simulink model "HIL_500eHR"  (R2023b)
settings: Solver=VariableStepAuto  StartTime=0.0  StopTime=Time  RelTol=1e-3
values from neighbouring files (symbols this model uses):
  BEV_mot = load("20241002_EM_Polito_Maps.mat")    [Init_FWD_500eHR.m]
undefined symbols (not defined in the file or in its folder): battery350V, bevGear, flip, motorDrive, T_EM_max, T_EM_max_cont, vehicle
libraries: fl_lib x38, nesl_utility x25, sdl_lib x11, slpidlib x3, simulink x3, ee_lib x2
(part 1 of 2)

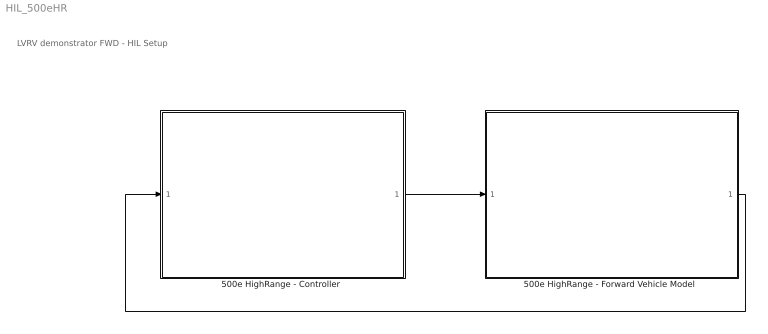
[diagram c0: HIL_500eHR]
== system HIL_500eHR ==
  note: LVRV demonstrator FWD - HIL Setup
  "500e HighRange - Controller " : Subsystem
  "500e HighRange - Forward Vehicle Model " : Subsystem
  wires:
  "500e HighRange - Forward Vehicle Model "/1(Bus Element Out) -> "500e HighRange - Controller "/1(BusElementIn)
  "500e HighRange - Controller "/1(Bus Element Out) -> "500e HighRange - Forward Vehicle Model "/1(BusElementIn)

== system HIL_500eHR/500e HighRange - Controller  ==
  BusElementIn : Inport
  BusElementIn1 : Inport
  Longitudinal Driver : Subsystem
  Memory : Memory  InheritSampleTime=on
  Memory1 : Memory  InheritSampleTime=on
  Terminator : Terminator
  Bus Element Out : Outport
  BusElementOut1 : Outport
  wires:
  Longitudinal Driver/2(BrakeCmd) -> Bus Element Out/1
  Memory/1 -> Longitudinal Driver/1(VehSpeed)
  Memory1/1 -> Terminator/1
  BusElementIn/1 -> Memory/1
  Longitudinal Driver/1(TorqueCmd) -> BusElementOut1/1
  BusElementIn1/1 -> Memory1/1

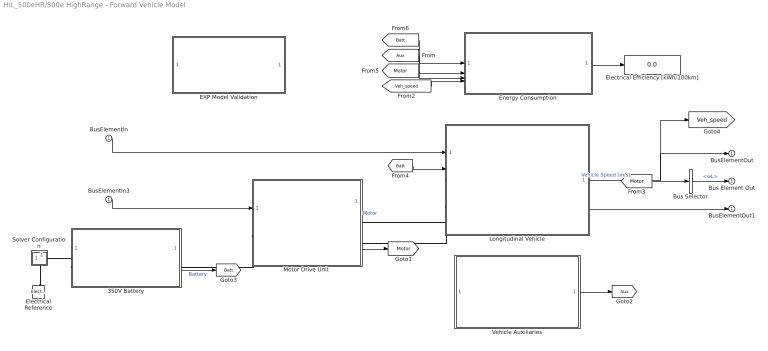
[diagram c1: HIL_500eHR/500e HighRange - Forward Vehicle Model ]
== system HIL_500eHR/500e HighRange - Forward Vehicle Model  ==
  BusElementIn : Inport
  BusElementIn3 : Inport
  350V Battery : Subsystem
  Bus Selector : BusSelector  OutputSignals=wL
  EXP Model Validation : Subsystem  Commented=on
  Electrical Reference : fl_lib/Electrical/Electrical Elements/Electrical Reference
  Electrical Efficiency [kWh/100km] : Display
  Energy Consumption : Subsystem
  Longitudinal Vehicle : Subsystem
  "Motor Drive Unit " : Subsystem
  Solver Configuration : Subsystem
  Vehicle Auxiliaries : Subsystem
  Bus Element Out : Outport
  BusElementOut : Outport
  BusElementOut1 : Outport
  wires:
  [Veh_speed] -> Energy Consumption/4(Veh_speed)
  Longitudinal Vehicle/2(Vehicle_Acceleration [m/s]) -> BusElementOut1/1
  BusElementIn/1 -> Longitudinal Vehicle/1(BrakeCtrl)
  [Motor] -> Bus Selector/1
  BusElementIn3/1 -> "Motor Drive Unit "/1(Input)
  [Batt] -> Longitudinal Vehicle/2(In Bus Element)
  Vehicle Auxiliaries/1(AuxPwr) -> [Aux]
  Bus Selector/1 -> Bus Element Out/1  "<wL>"
  [Motor] -> Energy Consumption/3(In Bus Element5)
  Longitudinal Vehicle/1(Vehicle_Velocity [m/s]) -> [Veh_speed], BusElementOut/1  "Vehicle Speed [m/s]"
  Energy Consumption/1(ElecEff) -> Electrical Efficiency [kWh/100km]/1
  [Batt] -> Energy Consumption/1(In Bus Element3)
  "Motor Drive Unit "/1(Bus Element Out) -> [Motor]  "Motor"
  [Aux] -> Energy Consumption/2(Loads)
  350V Battery/1(Info) -> [Batt]  "Battery"
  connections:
  "Motor Drive Unit "/LConn1 -- 350V Battery/RConn1
  Longitudinal Vehicle/LConn1 -- "Motor Drive Unit "/RConn1
  350V Battery/LConn1 -- Solver Configuration/RConn1
  Longitudinal Vehicle/LConn2 -- "Motor Drive Unit "/RConn2
  Electrical Reference/LConn1 -- Solver Configuration/RConn2

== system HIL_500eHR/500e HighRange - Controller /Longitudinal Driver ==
  note: 0 - 100 km/h time
  VehSpeed : Inport  Unit=m/s
  Constant : Constant  Value=0
  Drive cycle : Subsystem
  Manual Switch : ManualSwitch
  PI Driver : Subsystem
  Ramp : simulink/Sources/Ramp  slope=10  start=0  InitialOutput=0
  Saturation : Saturate  UpperLimit=130/3.6  LowerLimit=0
  Torque Distribution OnePedal : Subsystem
  TorqueCmd : Outport  Unit=N*m
  BrakeCmd : Outport  Port=2  Unit=Pa
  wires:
  Torque Distribution OnePedal/1(TrqCmd) -> TorqueCmd/1  "TorqueCmd"
  Torque Distribution OnePedal/2(BrakeCmd) -> BrakeCmd/1  "BrakeCmd"
  Ramp/1 -> Saturation/1
  Saturation/1 -> Manual Switch/1
  VehSpeed/1 -> PI Driver/2(Feedback)
  PI Driver/1(Command) -> Torque Distribution OnePedal/1(Required Torque)  "Torque Command"
  Constant/1 -> Manual Switch/2
  Drive cycle/1(V_ref) -> PI Driver/1(Reference)

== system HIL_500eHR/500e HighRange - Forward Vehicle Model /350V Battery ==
  note: High Voltage Battery
  350V Battery Status : Subsystem
  Auxiliaries load : fl_lib/Electrical/Electrical Elements/Resistor  R=(battery350V.nominalVoltage_V^2)/250 Ohm  i_specify=off  i_priority=None  i=0 A  i_nominal_specify=off  i_nominal_unit=A  i_nominal_value=1  v_specify=off  v_priority=None  v=0 V  v_nominal_specify=off  v_nominal_unit=V  v_nominal_value=1
  Current Sensor : fl_lib/Electrical/Electrical Sensors/Current Sensor
  DC Voltage Source : fl_lib/Electrical/Electrical Sources/DC Voltage Source  v0=battery350V.nominalVoltage_V V
  Internal Resistance : fl_lib/Electrical/Electrical Elements/Resistor  R=battery350V.internalResistance_Ohm Ohm  i_specify=off  i_priority=High  i=0 A  i_nominal_specify=off  i_nominal_unit=A  i_nominal_value=1  v_specify=off  v_priority=High  v=0 V  v_nominal_specify=off  v_nominal_unit=V  v_nominal_value=1
  Simscape Bus : SimscapeBus  HierarchyStrings=plus;minus
  Subsystem2 : Subsystem
  Voltage Sensor : fl_lib/Electrical/Electrical Sensors/Voltage Sensor
  GND : PMIOPort  Side=Left
  350V : PMIOPort  Port=2  Side=Right
  Info : Outport
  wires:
  350V Battery Status/1(Out Bus Element) -> Info/1, [Info]
  [Info] -> Subsystem2/1(In1)
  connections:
  Internal Resistance/RConn1 -- Auxiliaries load/RConn1 -- Current Sensor/LConn1
  Current Sensor/RConn2 -- Simscape Bus/LConn1 -- Voltage Sensor/LConn1
  350V Battery Status/LConn1 -- Voltage Sensor/RConn1
  DC Voltage Source/LConn1 -- Auxiliaries load/LConn1 -- Internal Resistance/LConn1
  350V Battery Status/LConn2 -- Current Sensor/RConn1
  DC Voltage Source/RConn1 -- GND/RConn1 -- Simscape Bus/LConn2 -- Voltage Sensor/RConn2
  350V/RConn1 -- Simscape Bus/RConn1

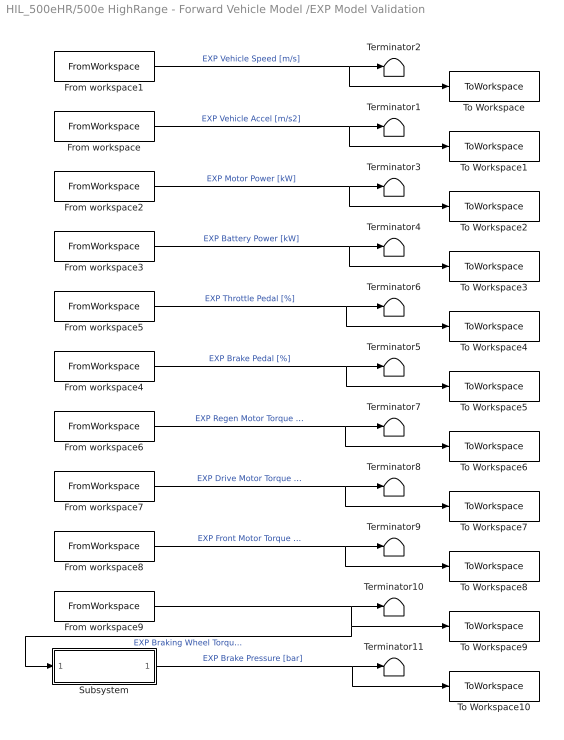
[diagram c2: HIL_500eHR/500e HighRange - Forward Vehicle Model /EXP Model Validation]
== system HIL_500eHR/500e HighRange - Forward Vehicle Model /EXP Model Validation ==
  From workspace : FromWorkspace  VariableName=aveh  SampleTime=0.1
  From workspace1 : FromWorkspace  VariableName=Vveh  SampleTime=0.1
  From workspace2 : FromWorkspace  VariableName=Pmot  SampleTime=0.1
  From workspace3 : FromWorkspace  VariableName=Pbatt  SampleTime=0.1
  From workspace4 : FromWorkspace  VariableName=BrkPedal  SampleTime=0.1
  From workspace5 : FromWorkspace  VariableName=GasPedal  SampleTime=0.1
  From workspace6 : FromWorkspace  VariableName=Treg  SampleTime=0.1
  From workspace7 : FromWorkspace  VariableName=Tdrive  SampleTime=0.1
  From workspace8 : FromWorkspace  VariableName=Tfront  SampleTime=0.1
  From workspace9 : FromWorkspace  VariableName=Tbrake  SampleTime=0.1
  Subsystem : Subsystem
  Terminator{1..11} (11 alike) : Terminator
  To Workspace : ToWorkspace  VariableName=Vveh  SampleTime=0.1
  To Workspace1 : ToWorkspace  VariableName=aveh  SampleTime=0.1
  To Workspace10 : ToWorkspace  VariableName=pbrake  SampleTime=0.1
  To Workspace2 : ToWorkspace  VariableName=Pmot  SampleTime=0.1
  To Workspace3 : ToWorkspace  VariableName=Pbatt  SampleTime=0.1
  To Workspace4 : ToWorkspace  VariableName=GasPedal  SampleTime=0.1
  To Workspace5 : ToWorkspace  VariableName=BrkPedal  SampleTime=0.1
  To Workspace6 : ToWorkspace  VariableName=Treg  SampleTime=0.1
  To Workspace7 : ToWorkspace  VariableName=Tdrive  SampleTime=0.1
  To Workspace8 : ToWorkspace  VariableName=Tfront  SampleTime=0.1
  To Workspace9 : ToWorkspace  VariableName=Tbrake  SampleTime=0.1
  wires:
  From workspace/1 -> To Workspace1/1, Terminator1/1  "EXP Vehicle Accel [m/s2]"
  From workspace1/1 -> To Workspace/1, Terminator2/1  "EXP Vehicle Speed [m/s]"
  From workspace2/1 -> To Workspace2/1, Terminator3/1  "EXP Motor Power [kW]"
  From workspace3/1 -> To Workspace3/1, Terminator4/1  "EXP Battery Power [kW]"
  From workspace7/1 -> To Workspace7/1, Terminator8/1  "EXP Drive Motor Torque [Nm]"
  From workspace6/1 -> To Workspace6/1, Terminator7/1  "EXP Regen Motor Torque [Nm]"
  From workspace5/1 -> To Workspace4/1, Terminator6/1  "EXP Throttle Pedal [%]"
  From workspace4/1 -> To Workspace5/1, Terminator5/1  "EXP Brake Pedal [%]"
  From workspace8/1 -> To Workspace8/1, Terminator9/1  "EXP Front Motor Torque [Nm]"
  From workspace9/1 -> Subsystem/1(Tb [Nm]), To Workspace9/1, Terminator10/1  "EXP Braking Wheel Torque [Nm]"
  Subsystem/1(pb [bar]) -> To Workspace10/1, Terminator11/1  "EXP Brake Pressure [bar]"

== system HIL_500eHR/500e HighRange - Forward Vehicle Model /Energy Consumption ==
  In Bus Element{1,3,7..8} (4 alike) : Inport
  Loads : Inport  Port=2
  In Bus Element6 : Inport  Port=3
  In Bus Element5 : Inport  Port=3
  Veh_speed : Inport  Port=4
  Electrical Efficiency : Subsystem
  Gain : Gain  Gain=3.6
  Scope Battery : Scope  NumInputPorts=4
  Scope Vehicle : Scope  NumInputPorts=3
  ElecEff : Outport
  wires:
  In Bus Element1/1 -> Scope Battery/3  "Battery Charge [Ah]"
  In Bus Element3/1 -> Scope Battery/1  "Battery Current [A]"
  In Bus Element5/1 -> Scope Vehicle/2  "Motor speed [rpm]"
  In Bus Element6/1 -> Scope Vehicle/3  "Motor Torque Command [Nm]"
  In Bus Element8/1 -> Scope Battery/2  "Battery Voltage [V]"
  Electrical Efficiency/1(ElecEff) -> ElecEff/1, Scope Battery/4  "Electrical Efficiency [kWh/100km]"
  In Bus Element7/1 -> Electrical Efficiency/2(BattPwr)  "Battery Power [kW]"
  Veh_speed/1 -> Gain/1
  Loads/1 -> Electrical Efficiency/1(AuxPwr)  "Auxiliaries Power [kW]"
  Gain/1 -> Scope Vehicle/1, Electrical Efficiency/3(VheSpd)  "Vehicle Speed [km/h]"

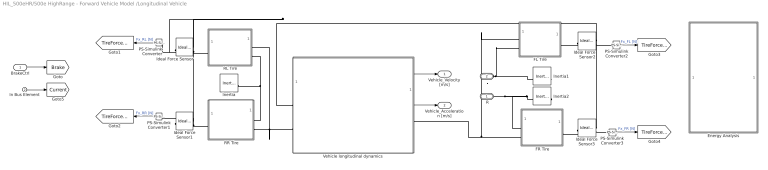
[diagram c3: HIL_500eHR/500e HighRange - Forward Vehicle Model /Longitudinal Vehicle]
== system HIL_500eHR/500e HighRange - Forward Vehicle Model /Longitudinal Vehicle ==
  BrakeCtrl : Inport
  In Bus Element : Inport  Port=2
  Energy Analysis : Subsystem  Commented=on
  FL Tire : Subsystem
  FR Tire : Subsystem
  Ideal Force Sensor{,1..3} (4 alike) : fl_lib/Mechanical/Mechanical Sensors/Ideal Force Sensor
  Inertia : fl_lib/Mechanical/Rotational Elements/Inertia  inertia=0.01 kg*m^2  num_ports=foundation.enum.numPorts2.one  w_specify=off  w_priority=High  w=0 rad/s  w_nominal_specify=off  w_nominal_unit=rad/s  w_nominal_value=1  t_specify=off  t_priority=None  t=0 N*m  t_nominal_specify=off  t_nominal_unit=N*m  t_nominal_value=1
  Inertia1 : fl_lib/Mechanical/Rotational Elements/Inertia  inertia=0.01 kg*m^2  num_ports=foundation.enum.numPorts2.one  w_specify=off  w_priority=High  w=0 rad/s  w_nominal_specify=off  w_nominal_unit=rad/s  w_nominal_value=1  t_specify=off  t_priority=None  t=0 N*m  t_nominal_specify=off  t_nominal_unit=N*m  t_nominal_value=1
  Inertia2 : fl_lib/Mechanical/Rotational Elements/Inertia  inertia=0.01 kg*m^2  num_ports=foundation.enum.numPorts2.one  w_specify=off  w_priority=High  w=0 rad/s  w_nominal_specify=off  w_nominal_unit=rad/s  w_nominal_value=1  t_specify=off  t_priority=None  t=0 N*m  t_nominal_specify=off  t_nominal_unit=N*m  t_nominal_value=1
  PS-Simulink Converter{,1..3} (4 alike) : nesl_utility/PS-Simulink Converter  PhysicalDomain=network_engine_domain  SubClassName=ps_output  LeftPortType=input  RightPortType=output  PseudoPeriodic=off  Frequencies=[]  VectorFormat=inherit  Unit=N  AffineConversion=off
  RL Tire : Subsystem
  RR Tire : Subsystem
  Vehicle longitudinal dynamics : Subsystem
  " R" : PMIOPort  Side=Left
  " L" : PMIOPort  Port=2  Side=Left
  Vehicle_Velocity [m/s] : Outport  VectorParamsAs1DForOutWhenUnconnected=off
  Vehicle_Acceleration [m/s] : Outport  Port=2  VectorParamsAs1DForOutWhenUnconnected=off
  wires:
  BrakeCtrl/1 -> [Brake]
  PS-Simulink Converter/1 -> [TireForce_RL]  "Fx_RL [N]"
  PS-Simulink Converter1/1 -> [TireForce_RR]  "Fx_RR [N]"
  PS-Simulink Converter2/1 -> [TireForce_FL]  "Fx_FL [N]"
  PS-Simulink Converter3/1 -> [TireForce_FR]  "Fx_FR [N]"
  In Bus Element/1 -> [Current]
  Vehicle longitudinal dynamics/1(V_act) -> Vehicle_Velocity [m/s]/1
  Vehicle longitudinal dynamics/2(a_act) -> Vehicle_Acceleration [m/s]/1
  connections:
  " L"/RConn1 -- Inertia1/LConn1 -- FL Tire/LConn2
  RR Tire/LConn2 -- Vehicle longitudinal dynamics/LConn2 -- RL Tire/LConn1
  Inertia2/LConn1 -- " R"/RConn1 -- FR Tire/LConn1
  Inertia/LConn1 -- RR Tire/LConn1 -- RL Tire/LConn2
  FR Tire/LConn2 -- Vehicle longitudinal dynamics/RConn1 -- FL Tire/LConn1
  Ideal Force Sensor3/RConn1 -- Ideal Force Sensor1/RConn1 -- Ideal Force Sensor/RConn1 -- Vehicle longitudinal dynamics/LConn1 -- Ideal Force Sensor2/RConn1
  Ideal Force Sensor/LConn1 -- RL Tire/RConn1
  PS-Simulink Converter2/LConn1 -- Ideal Force Sensor2/RConn2
  PS-Simulink Converter3/LConn1 -- Ideal Force Sensor3/RConn2
  Ideal Force Sensor1/LConn1 -- RR Tire/RConn1
  Ideal Force Sensor2/LConn1 -- FL Tire/RConn1
  Ideal Force Sensor3/LConn1 -- FR Tire/RConn1
  Ideal Force Sensor1/RConn2 -- PS-Simulink Converter1/LConn1
  PS-Simulink Converter/LConn1 -- Ideal Force Sensor/RConn2

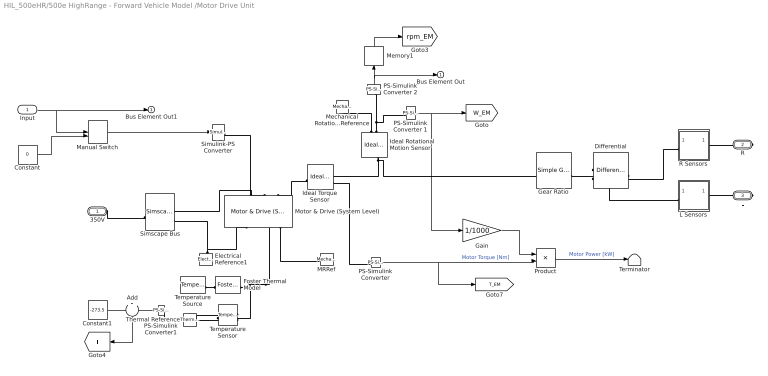
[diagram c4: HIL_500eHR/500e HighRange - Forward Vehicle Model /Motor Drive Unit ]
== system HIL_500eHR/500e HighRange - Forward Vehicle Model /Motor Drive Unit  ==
  Input : Inport
  " Simscape Bus" : SimscapeBus  HierarchyStrings=plus;minus
  Add : Sum
  Constant : Constant  Value=0
  Constant1 : Constant  Value=-273.5
  Differential : sdl_lib/Gears/Differential  driveshaft_location=sdl.enum.differential_orientation.right  cd_ratio=1  friction_model=sdl.enum.gear_friction.none  efficiency=[.85, .92]  temperature_TLU=[280, 300, 320] K  efficiency_ss_TLU=[.95, .9, .85]  efficiency_cd_TLU=[.95, .9, .85]  pwr_thr=[.001, .001] W  mu_visc=[0, 0] N*m*s/rad  model_inertia=simscape.enum.onoff.off  carrier_inertia=0.001 kg*m^2  planet_inertia=0.001 kg*m^2  thermal_mass=50 J/K  T_init=300 K
  Electrical Reference1 : fl_lib/Electrical/Electrical Elements/Electrical Reference
  Foster Thermal Model : ee_lib/Passive/Thermal/Foster Thermal Model  resistance_data=[0.079] K/W  tau_data=[51] s  steadyState=simscape.enum.onoff.on  Tvec_specify=off  Tvec_priority=None  Tvec=[300, 300, 300, 300] K  Tvec_nominal_specify=off  Tvec_nominal_unit=K  Tvec_nominal_value=1  Q_specify=off  Q_priority=None  Q=0 W  Q_nominal_specify=off  Q_nominal_unit=W  Q_nominal_value=1
  Gain : Gain  Gain=1/1000
  Gear Ratio : sdl_lib/Gears/Simple Gear  ratio=bevGear.gearRatio  rotation_direction=sdl.enum.shaftOutputDirection.same  friction_model=sdl.enum.gear_efficiencies_load.constant  T_noload=0.1 N*m  T_nom=5 N*m  efficiency_nom=0.8  efficiency=bevGear.efficiency  temperature_TLU=[280, 300, 320] K  load_TLU=[1, 5, 10] N*m  efficiency_TLU=[.95, .9, .85]  efficiency_TLU2=[.85, .8, .75; .95, .9, .85; .85, .8, .7]  w_thr=0.01 rad/s  pwr_thr=0.001 W  enable_backlash=false  hardstop_model=simscape.enum.hardstop.smooth  backlash_distance=1e-3 mm  r_base=0.1 m  transition=1e-4 mm  backlash_stiffness=1e7 N/m  backlash_damping=1e6 N*s/m  coeff_rest=0  v_tol=0.001 m/s  f_tol=0 N  mu_visc=[0, 0] N*m*s/rad  enable_faults=simscape.enum.onoff.off  efficiency_fault=0.05  external_fault=simscape.enum.onoff.off  temporal_fault=simscape.enum.onoff.off  fault_time=5 s  fault_angles=pi / 12 rad  report_fault=simscape.enum.assert.action.none  thermal_mass=50 J/K  temperature_specify=off  temperature_priority=High  temperature=300 K  temperature_nominal_specify=off  temperature_nominal_unit=K  temperature_nominal_value=1  x_backlash_specify=off  x_backlash_priority=None  x_backlash=0 mm  x_backlash_nominal_specify=off  x_backlash_nominal_unit=mm  x_backlash_nominal_value=1  f_hardstop_specify=off  f_hardstop_priority=None  f_hardstop=0 N  f_hardstop_nominal_specify=off  f_hardstop_nominal_unit=N  f_hardstop_nominal_value=1  v_backlash_specify=off  v_backlash_priority=None  v_backlash=0 m/s  v_backlash_nominal_specify=off  v_backlash_nominal_unit=m/s  v_backlash_nominal_value=1
  Ideal Rotational Motion Sensor : fl_lib/Mechanical/Mechanical Sensors/Ideal Rotational Motion Sensor  reference=foundation.enum.MeasurementReference.difference  acceleration_port=false  velocity_port=true  position_port=true  wrap_angle=false  offset=0 rad
  Ideal Torque Sensor : fl_lib/Mechanical/Mechanical Sensors/Ideal Torque Sensor
  L Sensors : Subsystem
  MRRef : fl_lib/Mechanical/Rotational Elements/Mechanical Rotational Reference
  Manual Switch : ManualSwitch
  Mechanical Rotational Reference : fl_lib/Mechanical/Rotational Elements/Mechanical Rotational Reference
  Memory1 : Memory  InheritSampleTime=on
  Motor & Drive (System Level) : ee_lib/Electromechanical/Motor & Drive (System Level)  torque_speed_param=ee.enum.electromech.envelope.tabulated  overtorque_param=ee.enum.electromech.overtorque.no  T_t=Shaft_Torque_max' N*m  T_t_intermittent=T_EM_max' N*m  T_t_2D=[T_EM_max_cont,T_EM_max_cont] N*m  T_t_intermittent_2D=[T_EM_max,T_EM_max] N*m  w_t=Speed_max' rpm  vdc_t=[48,52] V  torque_max=motorDrive.simplePmsmDrv_trqMax_Nm N*m  power_max=motorDrive.simplePmsmDrv_powMax_W W  torque_max_intermittent=0.4 N*m  power_max_intermittent=120 W  time_overtorque=60 s  time_recover=60 s  Tc=motorDrive.simplePmsmDrv_timeConst_s s  EnableSwitch=simscape.enum.onoff.off  losses_param=2  eff=100  w_eff=3750 rpm  T_eff=0.08 N*m  Piron=0 W  Pbase=0 W  w_eff_vec=BEV_mot.Speed(:,1)' rpm  T_eff_vec=flip(BEV_mot.Shaft_Torque(1,:)) N*m  v_eff_vec=[100, 250, 400] V  losses_mat=flip(BEV_mot.Total_Loss,2) W  efficiency_mat=eff_motor  losses_mat_3D=ones(5, 4, 3) W  efficiency_mat_3D=95 * ones(5, 4, 3)  Res=0 Ohm  enable_fault=simscape.enum.onoff.off  fault_condition=1  fault_threshold=0.5  J=motorDrive.simplePmsmDrv_rotorInertia_kg_m2 kg*m^2  lam=motorDrive.simplePmsmDrv_rotorDamping_Nm_per_radps N*m/(rad/s)  speed0=motorDrive.simplePmsmDrv_initialRotorSpd_rpm rpm  faulted_specify=off  faulted_priority=None  faulted=0  faulted_nominal_specify=off  faulted_nominal_unit=1  faulted_nominal_value=1  isSwitchedOff_specify=off  isSwitchedOff_priority=None  isSwitchedOff=0  isSwitchedOff_nominal_specify=off  isSwitchedOff_nominal_unit=1  isSwitchedOff_nominal_value=1  torqueLimitContinuous_specify=off  torqueLimitContinuous_priority=None  torqueLimitContinuous=0 N*m  torqueLimitContinuous_nominal_specify=off  torqueLimitContinuous_nominal_unit=N*m  torqueLimitContinuous_nominal_value=1  alpha=3.93e-3 1/K  Tmeas=298.5 K  Tmeas2=50+273.5 K  losses_mat_T2=flip(BEV_mot.Total_Loss,2) W  efficiency_mat_T2=[95, 95, 95, 95; 95, 95, 95, 95; 95, 95, 95, 95; 95, 95, 95, 95; 95, 95, 95, 95]  losses_mat_3D_T2=ones(5, 4, 3) W  efficiency_mat_3D_T2=95 * ones(5, 4, 3)  thermal_mass=0.0001 J/K  initial_temperature=298.5 K
  PS-Simulink Converter : nesl_utility/PS-Simulink Converter  PhysicalDomain=network_engine_domain  SubClassName=ps_output  LeftPortType=input  RightPortType=output  PseudoPeriodic=off  Frequencies=[]  VectorFormat=1-D array  Unit=N*m  AffineConversion=off
  PS-Simulink Converter 1 : nesl_utility/PS-Simulink Converter  PhysicalDomain=network_engine_domain  SubClassName=ps_output  LeftPortType=input  RightPortType=output  PseudoPeriodic=off  Frequencies=[]  VectorFormat=1-D array  Unit=rad/s  AffineConversion=off
  PS-Simulink Converter 2 : nesl_utility/PS-Simulink Converter  PhysicalDomain=network_engine_domain  SubClassName=ps_output  LeftPortType=input  RightPortType=output  PseudoPeriodic=off  Frequencies=[]  VectorFormat=1-D array  Unit=rpm  AffineConversion=off
  PS-Simulink Converter1 : nesl_utility/PS-Simulink Converter  PhysicalDomain=network_engine_domain  SubClassName=ps_output  LeftPortType=input  RightPortType=output  PseudoPeriodic=off  Frequencies=[]  VectorFormat=inherit  Unit=inherit  AffineConversion=off
  Product : Product
  R Sensors : Subsystem
  Simulink-PS Converter : nesl_utility/Simulink-PS Converter  PhysicalDomain=network_engine_domain  SubClassName=ps_input  LeftPortType=input  RightPortType=output  PseudoPeriodic=off  Frequencies=[]  NoiseDistribution=none  NoiseParameters=[]  Unit=N*m  AffineConversion=off  FilteringAndDerivatives=zero  SimscapeFilterOrder=1  InputFilterTimeConstant=.001  UdotUserProvided=0
  Temperature Sensor : fl_lib/Thermal/Thermal Sensors/Temperature Sensor  temperature_measure=foundation.enum.MeasurementReference.difference
  Temperature Source : fl_lib/Thermal/Thermal Sources/Temperature Source  temperature=273.15+40 K
  Terminator : Terminator
  Thermal Reference : fl_lib/Thermal/Thermal Elements/Thermal Reference
  350V : PMIOPort  Side=Left
  R : PMIOPort  Port=2  Side=Right
  L : PMIOPort  Port=3  Side=Right
  Bus Element Out : Outport
  Bus Element Out1 : Outport
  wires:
  Input/1 -> Manual Switch/1, Bus Element Out1/1
  PS-Simulink Converter/1 -> Product/2, [T_EM]  "Motor Torque [Nm]"
  Product/1 -> Terminator/1  "Motor Power [kW]"
  Gain/1 -> Product/1
  PS-Simulink Converter 1/1 -> [W_EM], Gain/1
  Constant/1 -> Manual Switch/2
  Memory1/1 -> [rpm_EM]
  Manual Switch/1 -> Simulink-PS Converter/1
  Add/1 -> [T]
  PS-Simulink Converter1/1 -> Add/2
  Constant1/1 -> Add/1
  PS-Simulink Converter 2/1 -> Bus Element Out/1, Memory1/1
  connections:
  Ideal Rotational Motion Sensor/LConn1 -- Gear Ratio/LConn1 -- Ideal Torque Sensor/RConn1
  Simulink-PS Converter/RConn1 -- Motor & Drive (System Level)/LConn2
  Ideal Rotational Motion Sensor/RConn1 -- Mechanical Rotational Reference/LConn1
  Motor & Drive (System Level)/LConn1 -- " Simscape Bus"/LConn1
  350V/RConn1 -- " Simscape Bus"/RConn1
  Electrical Reference1/LConn1 -- Motor & Drive (System Level)/RConn1 -- " Simscape Bus"/LConn2
  Ideal Rotational Motion Sensor/RConn2 -- PS-Simulink Converter 1/LConn1 -- PS-Simulink Converter 2/LConn1
  Ideal Torque Sensor/LConn1 -- Motor & Drive (System Level)/LConn3
  Ideal Torque Sensor/RConn2 -- PS-Simulink Converter/LConn1
  R Sensors/RConn1 -- R/RConn1
  R Sensors/LConn1 -- Differential/RConn2
  Differential/RConn1 -- L Sensors/LConn1
  L Sensors/RConn1 -- L/RConn1
  Differential/LConn1 -- Gear Ratio/RConn1
  Motor & Drive (System Level)/RConn4 -- MRRef/LConn1
  Foster Thermal Model/LConn1 -- Temperature Sensor/LConn1 -- Motor & Drive (System Level)/RConn3
  PS-Simulink Converter1/LConn1 -- Temperature Sensor/RConn2
  Thermal Reference/LConn1 -- Temperature Sensor/RConn1
  Foster Thermal Model/RConn1 -- Temperature Source/LConn1

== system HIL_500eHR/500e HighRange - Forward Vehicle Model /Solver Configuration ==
  note: Simscape needs a Solver Configuration block per physical network.
  Solver Configuration : nesl_utility/Solver Configuration  PhysicalDomain=network_engine_domain  SubClassName=solver  LeftPortType=input  RightPortType=generic  Tones=[]  Harmonics=[]  SimulateNoise=off  Profile=off  UseLocalSampling=off  EnableSwitchedLinearOptims=on  FrequencyDomain=off  UseCCode=off  RelTol=0.001  AbsTol=1e-06  MinStep=1e-09  ToWorkspace=off  RevertToSquareIcSolve=off  NumHomotopyIterations=100  PhasorMode=off  PhasorModeNumHarmonics=1  ConsistencySolver=NEWTON_FTOL  IndexReductionMethod=DerivativeReplacement  DoDC=off  ResidualTolerance=1e-6  ConsistencyTolSource=GLOBAL  ConsistencyAbsTol=0.001  ConsistencyRelTol=0.001  ConsistencyTolFactor=0.001  UseLocalSolver=on  LocalSolverChoice=NE_BACKWARD_EULER_ADVANCER  ResolveIndetEquations=on  FunctionEvalNumThread=1  LocalSolverSampleTime=0.01  DoFixedCost=on  MaxNonlinIter=3  MaxModeIter=2  ComputeImpulses=off  ImpulseIterations=2  LinearAlgebra=auto  LinearAlgebraNumThread=0  EquationFormulation=NE_TIME_EF  DelaysMemoryBudget=1024  AutomaticFiltering=on  FilteringTimeConstant=0.001  PartitionStorageMethod=AS_NEEDED  PartitionMemoryBudget=1024  PartitionMethod=FAST  MultibodyUseLocalSolver=off  MultibodyLocalSolverChoice=ODE1  MultibodyLocalSolverSampleTime=0.001
  1 : PMIOPort  Side=Right
  2 : PMIOPort  Port=2  Side=Right
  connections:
  Solver Configuration/RConn1 -- 1/RConn1 -- 2/RConn1

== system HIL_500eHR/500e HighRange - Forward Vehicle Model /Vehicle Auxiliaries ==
  Constant Auxiliary Loads : Constant  Value=250
  Gain : Gain  Gain=1/1000
  AuxPwr : Outport
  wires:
  Gain/1 -> AuxPwr/1  "Auxiliaries Power [kW]"
  Constant Auxiliary Loads/1 -> Gain/1

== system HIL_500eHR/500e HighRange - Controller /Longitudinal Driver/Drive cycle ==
  From workspace : FromWorkspace  VariableName=Vveh  SampleTime=-1
  Gain : Gain  Gain=1.05
  Gain1 : Gain  Gain=0.95
  Terminator : Terminator
  Terminator1 : Terminator
  V_ref : Outport  VectorParamsAs1DForOutWhenUnconnected=off
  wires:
  Gain/1 -> Terminator/1  "Speed Ref Up [m/s]"
  Gain1/1 -> Terminator1/1  "Speed Ref Down [m/s]"
  From workspace/1 -> V_ref/1, Gain1/1, Gain/1  "Speed Reference [m/s]"

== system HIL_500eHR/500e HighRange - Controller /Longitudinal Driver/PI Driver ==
  Reference : Inport
  Feedback : Inport  Port=2
  Add : Sum  Inputs=|+-
  MATLAB Function : MATLAB Function  TreatAsAtomicUnit=on
  Max Torque : Gain  Gain=87
  PI Controller : slpidlib/PID Controller  Controller=PI  Form=Parallel  TimeDomain=Discrete-time  UseExternalTs=off  SampleTime=0.2  IntegratorMethod=Forward Euler  FilterMethod=Forward Euler  ControllerParametersSource=internal  P=0.5  I=0.5/16.67  UseKiTs=off  D=0.15  N=100  UseFilter=on  TunerSelectOption=Transfer Function Based (PID Tuner App)  InitialConditionSource=internal  InitialConditionForIntegrator=0  InitialConditionForFilter=0  DifferentiatorICPrevScaledInput=0  ExternalReset=falling  TrackingMode=off  Kt=1  LimitOutput=on  SatLimitsSource=internal  UpperSaturationLimit=1  LowerSaturationLimit=-1  LinearizeAsGain=on  AntiWindupMode=clamping  Kb=1  LimitIntegrator=off  UpperIntegratorSaturationLimit=inf  LowerIntegratorSaturationLimit=-inf  POutMin=[]  POutMax=[]  IOutMin=[]  IOutMax=[]  DOutMin=[]  DOutMax=[]  NOutMin=[]  NOutMax=[]  SumOutMin=[]  SumOutMax=[]  SaturationOutMin=[]  SaturationOutMax=[]  PParamMin=[]  PParamMax=[]  IParamMin=[]  IParamMax=[]  DParamMin=[]  DParamMax=[]  NParamMin=[]  NParamMax=[]  KbParamMin=[]  KbParamMax=[]  KtParamMin=[]  KtParamMax=[]  KbOutMin=[]  KbOutMax=[]  KtOutMin=[]  KtOutMax=[]  IntegratorOutMin=[]  IntegratorOutMax=[]  FilterOutMin=[]  FilterOutMax=[]  SumI1OutMin=[]  SumI1OutMax=[]  SumI2OutMin=[]  SumI2OutMax=[]  SumI3OutMin=[]  SumI3OutMax=[]  SumI4OutMin=[]  SumI4OutMax=[]  SumDOutMin=[]  SumDOutMax=[]  DifferentiatorOutMin=[]  DifferentiatorOutMax=[]  FilterDiffOutCoefMin=[]  FilterDiffOutCoefMax=[]  ReciprocalOutMin=[]  ReciprocalOutMax=[]  SumDenOutMin=[]  SumDenOutMax=[]  SumNumOutMin=[]  SumNumOutMax=[]  DivideOutMin=[]  DivideOutMax=[]  UdiffTsProdOutMin=[]  UdiffTsProdOutMax=[]  NTsProdOutMin=[]  NTsProdOutMax=[]  UintegralTsProdOutMin=[]  UintegralTsProdOutMax=[]  UngainTsProdOutMin=[]  UngainTsProdOutMax=[]  ClampingZeroOutDataTypeStr=Inherit: Inherit via back propagation  ClampingZeroOutMin=[]  ClampingZeroOutMax=[]  FilterDenConstantOutDataTypeStr=Inherit: Inherit via back propagation  FilterDenConstantOutMin=[]  FilterDenConstantOutMax=[]  PCopyOutDataTypeStr=Inherit: Inherit via back propagation  PCopyOutMin=[]  PCopyOutMax=[]  NCopyOutDataTypeStr=Inherit: Inherit via back propagation  NCopyOutMin=[]  NCopyOutMax=[]  IntegratorContinuousStateAttributes=''  IntegratorStateMustResolveToSignalObject=off  IntegratorRTWStateStorageClass=Auto  FilterContinuousStateAttributes=''  FilterStateMustResolveToSignalObject=off  FilterRTWStateStorageClass=Auto  ParallelPVariant=InternalParameters  IdealPVariant=Disabled  IVariant=InternalParameters  DVariant=Disabled  IntegratorVariant=Discrete  SatVariant=Enabled  AWVariant=DiscClampingParallel  PCopyVariant=Disabled  TRVariant=Disabled  FdbkBlocksVariant=Forward  IdealPFdbkVariant=Disabled  SatFdbkVariant=Disabled  DerivativeFilterVariant=Disabled  NVariant=Disabled  NCopyVariant=Disabled_SignalSpec  FilterICVariant=Disabled  IntegratorICVariant=InternalICs  ExternalResetVariant=ExternalReset  TRSumVariant=Passthrough  SumFdbkVariant=Disabled  SumVariant=Sum_PI  TsampFilterVariant=InternalTs  TsampNgainVariant=Passthrough  TsampIntegralVariant=Disabled_SignalSpec  ExternalSaturationOutDataTypeStr=Inherit: Same as second input
  Terminator : Terminator
  Command : Outport  VectorParamsAs1DForOutWhenUnconnected=off
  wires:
  Add/1 -> PI Controller/1  "Error"
  Max Torque/1 -> Command/1, MATLAB Function/1(ReqTorque)  "Treq FB"
  MATLAB Function/1(GasPedal) -> Terminator/1  "Gas Pedal [%]"
  Reference/1 -> PI Controller/2, Add/1
  Feedback/1 -> Add/2, MATLAB Function/2(Speed)
  PI Controller/1 -> Max Torque/1  "throttle FB"

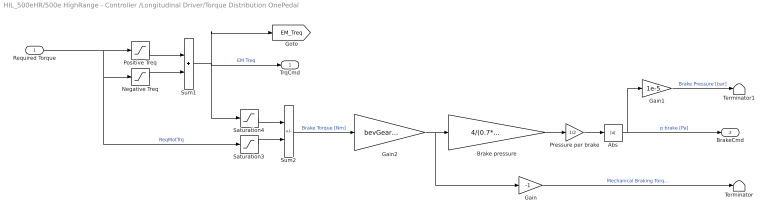
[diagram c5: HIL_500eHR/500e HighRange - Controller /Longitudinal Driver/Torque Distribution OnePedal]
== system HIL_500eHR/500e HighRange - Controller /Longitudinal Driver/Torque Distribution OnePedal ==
  Required Torque : Inport
  Abs : Abs
  Brake pressure : Gain  Gain=4/(0.7*pi*(0.025)^2*0.15*2)
  Gain : Gain  Gain=-1
  Gain1 : Gain  Gain=1e-5
  Gain2 : Gain  Gain=bevGear.gearRatio
  Negative Treq : Saturate  UpperLimit=0  LowerLimit=-87
  Positive Treq : Saturate  UpperLimit=87  LowerLimit=0
  Pressure per brake : Gain  Gain=1/2
  Saturation3 : Saturate  UpperLimit=0  LowerLimit=-inf
  Saturation4 : Saturate  UpperLimit=0  LowerLimit=-inf
  Sum1 : Sum
  Sum2 : Sum  Inputs=-+
  Terminator : Terminator
  Terminator1 : Terminator
  TrqCmd : Outport
  BrakeCmd : Outport  Port=2  Unit=Pa
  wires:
  Gain2/1 -> Gain/1, Brake pressure/1
  Pressure per brake/1 -> Abs/1
  Brake pressure/1 -> Pressure per brake/1
  Sum2/1 -> Gain2/1  "Brake Torque [Nm]"
  Abs/1 -> BrakeCmd/1, Gain1/1  "p brake [Pa]"
  Negative Treq/1 -> Sum1/2
  Positive Treq/1 -> Sum1/1
  Required Torque/1 -> Positive Treq/1, Saturation3/1, Negative Treq/1  "ReqMotTrq"
  Sum1/1 -> TrqCmd/1, [EM_Treq], Saturation4/1  "EM Treq"
  Saturation3/1 -> Sum2/2
  Saturation4/1 -> Sum2/1
  Gain/1 -> Terminator/1  "Mechanical Braking Torque [Nm]"
  Gain1/1 -> Terminator1/1  "Brake Pressure [bar]"

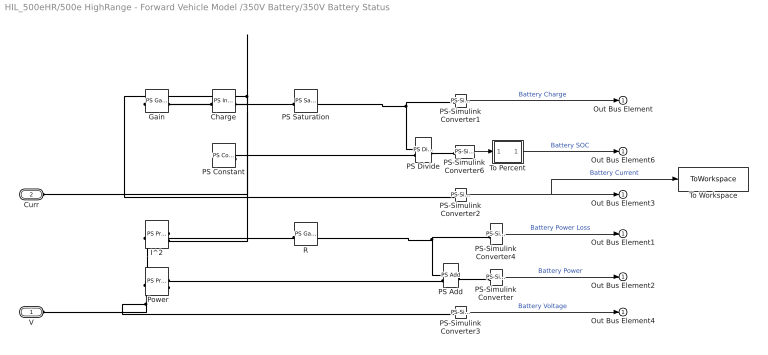
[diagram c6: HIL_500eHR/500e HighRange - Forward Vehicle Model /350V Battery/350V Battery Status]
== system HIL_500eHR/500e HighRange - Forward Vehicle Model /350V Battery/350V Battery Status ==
  Charge : fl_lib/Physical Signals/Linear Operators/PS Integrator  reset_method=foundation.enum.IntegratorResetSpec.None  initial_condition_spec=foundation.enum.IntegratorICSpec.Internal  saturation_spec=foundation.enum.IntegratorSaturationSpec.None  saturation_source_spec=foundation.enum.IntegratorSaturationSourceSpec.Internal  x0=initial.Battery_Charge_Ahr A*hr  xu=inf s  xl=-inf s
  Gain : fl_lib/Physical Signals/Functions/PS Gain  gain=-1
  I^2 : fl_lib/Physical Signals/Functions/PS Product
  PS Add : fl_lib/Physical Signals/Functions/PS Add
  PS Constant : fl_lib/Physical Signals/Sources/PS Constant  constant=battery350V.nominalCharge_Ahr A*hr
  PS Divide : fl_lib/Physical Signals/Functions/PS Divide
  PS Saturation : fl_lib/Physical Signals/Nonlinear Operators/PS Saturation  upper_limit=battery350V.nominalCharge_Ahr A*hr  lower_limit=0 A*hr
  PS-Simulink Converter : nesl_utility/PS-Simulink Converter  PhysicalDomain=network_engine_domain  SubClassName=ps_output  LeftPortType=input  RightPortType=output  PseudoPeriodic=off  Frequencies=[]  VectorFormat=1-D array  Unit=kW  AffineConversion=off
  PS-Simulink Converter1 : nesl_utility/PS-Simulink Converter  PhysicalDomain=network_engine_domain  SubClassName=ps_output  LeftPortType=input  RightPortType=output  PseudoPeriodic=off  Frequencies=[]  VectorFormat=1-D array  Unit=A*hr  AffineConversion=off
  PS-Simulink Converter2 : nesl_utility/PS-Simulink Converter  PhysicalDomain=network_engine_domain  SubClassName=ps_output  LeftPortType=input  RightPortType=output  PseudoPeriodic=off  Frequencies=[]  VectorFormat=1-D array  Unit=A  AffineConversion=off
  PS-Simulink Converter3 : nesl_utility/PS-Simulink Converter  PhysicalDomain=network_engine_domain  SubClassName=ps_output  LeftPortType=input  RightPortType=output  PseudoPeriodic=off  Frequencies=[]  VectorFormat=1-D array  Unit=V  AffineConversion=off
  PS-Simulink Converter4 : nesl_utility/PS-Simulink Converter  PhysicalDomain=network_engine_domain  SubClassName=ps_output  LeftPortType=input  RightPortType=output  PseudoPeriodic=off  Frequencies=[]  VectorFormat=1-D array  Unit=W  AffineConversion=off
  PS-Simulink Converter6 : nesl_utility/PS-Simulink Converter  PhysicalDomain=network_engine_domain  SubClassName=ps_output  LeftPortType=input  RightPortType=output  PseudoPeriodic=off  Frequencies=[]  VectorFormat=1-D array  Unit=1  AffineConversion=off
  Power : fl_lib/Physical Signals/Functions/PS Product
  R : fl_lib/Physical Signals/Functions/PS Gain  gain=battery350V.internalResistance_Ohm Ohm
  To Percent : Subsystem
  To Workspace : ToWorkspace  VariableName=Battery_current  SaveFormat=Timeseries  SampleTime=-1
  V : PMIOPort  Side=Left
  Curr : PMIOPort  Port=2  Side=Left
  Out Bus Element{,1..4,6} (6 alike) : Outport
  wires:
  PS-Simulink Converter6/1 -> To Percent/1(In1)
  To Percent/1(Out1) -> Out Bus Element6/1  "Battery SOC"
  PS-Simulink Converter3/1 -> Out Bus Element4/1  "Battery Voltage"
  PS-Simulink Converter2/1 -> To Workspace/1, Out Bus Element3/1  "Battery Current"
  PS-Simulink Converter4/1 -> Out Bus Element1/1  "Battery Power Loss"
  PS-Simulink Converter1/1 -> Out Bus Element/1  "Battery Charge"
  PS-Simulink Converter/1 -> Out Bus Element2/1  "Battery Power"
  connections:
  PS-Simulink Converter6/LConn1 -- PS Divide/RConn1
  Power/RConn1 -- PS Add/LConn2
  PS Constant/RConn1 -- PS Divide/LConn2
  PS Add/RConn1 -- PS-Simulink Converter/LConn1
  R/LConn1 -- I^2/RConn1
  PS Saturation/LConn1 -- Charge/RConn1
  Gain/RConn1 -- Charge/LConn1
  PS Add/LConn1 -- PS-Simulink Converter4/LConn1 -- R/RConn1
  Power/LConn1 -- V/RConn1 -- PS-Simulink Converter3/LConn1
  PS Divide/LConn1 -- PS Saturation/RConn1 -- PS-Simulink Converter1/LConn1
  Power/LConn2 -- I^2/LConn1 -- PS-Simulink Converter2/LConn1 -- Curr/RConn1 -- Gain/LConn1 -- I^2/LConn2

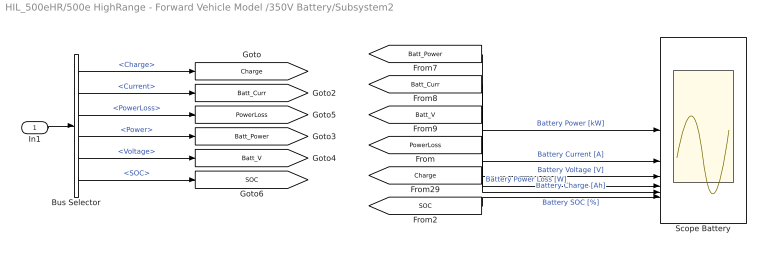
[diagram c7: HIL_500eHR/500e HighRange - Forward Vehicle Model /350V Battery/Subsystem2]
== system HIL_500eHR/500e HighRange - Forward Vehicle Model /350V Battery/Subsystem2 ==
  In1 : Inport
  Bus Selector : BusSelector  OutputSignals=Charge,Current,PowerLoss,Power,Voltage,SOC
  Scope Battery : Scope  NumInputPorts=6
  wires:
  Bus Selector/4 -> [Batt_Power]  "<Power>"
  [SOC] -> Scope Battery/6  "Battery SOC [%]"
  Bus Selector/6 -> [SOC]  "<SOC>"
  [Batt_V] -> Scope Battery/3  "Battery Voltage [V]"
  Bus Selector/3 -> [PowerLoss]  "<PowerLoss>"
  Bus Selector/1 -> [Charge]  "<Charge>"
  Bus Selector/2 -> [Batt_Curr]  "<Current>"
  [Charge] -> Scope Battery/5  "Battery Charge [Ah]"
  [Batt_Curr] -> Scope Battery/2  "Battery Current [A]"
  [Batt_Power] -> Scope Battery/1  "Battery Power [kW]"
  Bus Selector/5 -> [Batt_V]  "<Voltage>"
  [PowerLoss] -> Scope Battery/4  "Battery Power Loss [W]"
  In1/1 -> Bus Selector/1

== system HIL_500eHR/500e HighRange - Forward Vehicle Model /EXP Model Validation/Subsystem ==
  Tb [Nm] : Inport
  Abs : Abs
  Brake pressure : Gain  Gain=2/(0.7*pi*(0.025)^2*0.15*2)
  Gain1 : Gain  Gain=1e-5
  Pressure per brake : Gain  Gain=1/2
  pb [bar] : Outport
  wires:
  Tb [Nm]/1 -> Brake pressure/1
  Abs/1 -> Gain1/1  "p brake [Pa]"
  Brake pressure/1 -> Pressure per brake/1
  Gain1/1 -> pb [bar]/1  "EXP Brake Pressure [bar]"
  Pressure per brake/1 -> Abs/1

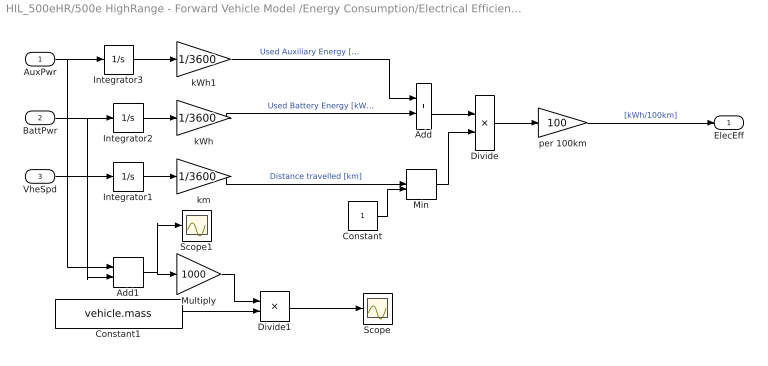
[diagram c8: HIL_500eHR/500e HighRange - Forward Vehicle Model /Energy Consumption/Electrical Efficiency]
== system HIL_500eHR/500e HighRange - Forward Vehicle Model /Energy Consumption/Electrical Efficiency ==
  AuxPwr : Inport
  BattPwr : Inport  Port=2  Unit=kW
  VheSpd : Inport  Port=3  Unit=km/hr
  Add : Sum
  Add1 : Sum
  Constant : Constant
  Constant1 : Constant  Value=vehicle.mass
  Divide : Product  Inputs=*/
  Divide1 : Product  Inputs=*/
  Integrator1 : Integrator
  Integrator2 : Integrator
  Integrator3 : Integrator
  Min : MinMax  Function=max  Inputs=2
  Multiply : Gain  Gain=1000
  Scope : Scope
  Scope1 : Scope
  kWh : Gain  Gain=1/3600
  kWh1 : Gain  Gain=1/3600
  km : Gain  Gain=1/3600
  per 100km : Gain  Gain=100
  ElecEff : Outport  Unit=kW*hr/km
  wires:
  km/1 -> Min/1  "Distance travelled [km]"
  Constant/1 -> Min/2
  Integrator2/1 -> kWh/1
  Divide/1 -> per 100km/1
  Integrator1/1 -> km/1
  Min/1 -> Divide/2
  kWh/1 -> Add/2  "Used Battery Energy [kWh]"
  per 100km/1 -> ElecEff/1  "[kWh/100km]"
  BattPwr/1 -> Add1/2, Integrator2/1
  VheSpd/1 -> Integrator1/1
  Add/1 -> Divide/1
  kWh1/1 -> Add/1  "Used Auxiliary Energy [kWh]"
  Integrator3/1 -> kWh1/1
  AuxPwr/1 -> Add1/1, Integrator3/1
  Constant1/1 -> Divide1/2
  Divide1/1 -> Scope/1
  Add1/1 -> Scope1/1, Multiply/1
  Multiply/1 -> Divide1/1

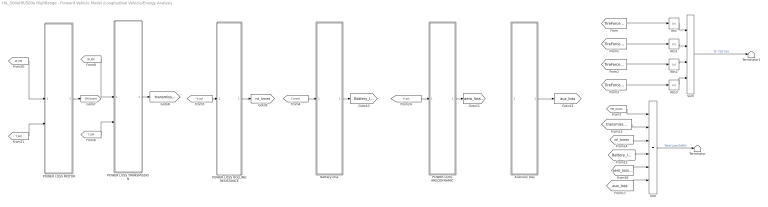
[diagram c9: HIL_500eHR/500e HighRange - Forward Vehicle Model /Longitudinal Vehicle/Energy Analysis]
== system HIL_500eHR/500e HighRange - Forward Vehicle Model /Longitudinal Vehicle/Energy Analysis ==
  Abs{,1..3} (4 alike) : Abs
  Add : Sum  Inputs=++++++
  Auxiliary loss : Subsystem
  Battery loss : Subsystem
  POWER LOSS AREODYNAMIC : Subsystem
  POWER LOSS MOTOR : Subsystem
  POWER LOSS ROLLING RESISTANCE : Subsystem
  POWER LOSS TRANSMISSION : Subsystem
  Sum : Sum  Inputs=++++
  Terminator : Terminator
  Terminator1 : Terminator
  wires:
  [T_EM] -> POWER LOSS MOTOR/2(T_EM)
  [TireForce_FL] -> Abs/1
  Abs3/1 -> Sum/4
  Abs/1 -> Sum/1
  Battery loss/1(Battery en. losses) -> [Battery_losses]
  [EM_losses] -> Add/1
  [TireForce_RR] -> Abs3/1
  [transmission_loss] -> Add/2
  [W_EM] -> POWER LOSS TRANSMISSION/1(W_EM)
  [aux_loss] -> Add/6
  POWER LOSS AREODYNAMIC/1(aero en. losses) -> [aero_losses]
  [TireForce_FR] -> Abs1/1
  [Battery_losses] -> Add/4
  [rol_losses] -> Add/3
  [T_EM] -> POWER LOSS TRANSMISSION/2(T_EM)
  [TireForce_RL] -> Abs2/1
  Abs2/1 -> Sum/3
  Sum/1 -> Terminator1/1  "TF_TOT [N]"
  Auxiliary loss/1(auxiliary en. loss) -> [aux_loss]
  Abs1/1 -> Sum/2
  [Current] -> Battery loss/1(Battery_I)
  POWER LOSS ROLLING RESISTANCE/1(Out1) -> [rol_losses]
  POWER LOSS TRANSMISSION/1(Transmission en loss) -> [transmission_loss]
  POWER LOSS MOTOR/1(EM en loss) -> [EM_losses]
  [aero_losses] -> Add/5
  [W_EM] -> POWER LOSS MOTOR/1(W_EM)
  [V_act] -> POWER LOSS AREODYNAMIC/1(v_act)
  Add/1 -> Terminator/1  "Total Loss [kWh]"
  [V_act] -> POWER LOSS ROLLING RESISTANCE/1(V act)

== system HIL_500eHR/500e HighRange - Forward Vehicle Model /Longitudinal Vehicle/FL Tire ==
  Disc Brake1 : sdl_lib/Brakes & Detents/Rotational/Disc Brake  r_mean=150 mm  bore=10 mm  n_pads=2  thermal_port=simscape.enum.thermaleffects.omit  mu_static=0.9  mu_coulomb=0.7  temperature_TLU=[280, 300, 320] K  mu_static_TLU=[.9, .8, .7]  mu_coulomb_TLU=[.8, .7, .6]  brkwy_vel=0.1 rad/s  visc_coef=.001 N*m/(rad/s)  enable_faults=simscape.enum.onoff.off  faulted_pressure=0 bar  external_fault=simscape.enum.onoff.off  temporal_fault=simscape.enum.onoff.off  fault_time=5 s  report_fault=simscape.enum.assert.action.none  thermal_mass=50 kJ/K  temperature_specify=off  temperature_priority=High  temperature=300 K  temperature_nominal_specify=off  temperature_nominal_unit=K  temperature_nominal_value=1
  FL Tire : sdl_lib/Tires & Vehicles/Tire (Magic Formula)  parameterization=sdl.enum.magic_tire_model.peak  F_z1=vehicle.mass*9.81/4 N  F_x1=3500 N  kappa1=10  B_m=14.2649  C_m=2.9817  D_m=0.7035  E_m=1.5923  fz0=4000 N  p_Cx=1.685  p_Dx=[1.21, -.037]  p_Ex=[.344, .095, -.02, 0]  p_Kx=[21.51, -.163, .245]  p_Hx=[-.002, .002]  p_Vx=[0, 0]  rolling_radius_model=sdl.enum.RollingRadiusParameterization.Constant  r_e=vehicle.tireRollingRadius m  r_0=0.3 m  breff=8.39  dreff=0.26  freff=0.074  q_re0=0.99  q_v1=0.008  longvl=17 m/s  cz=5e5 N/m  model_resistance=simscape.enum.onoff.on  resistance_model=sdl.enum.rollingResistanceParameterization.constant  coeff=vehicle.tireRRcoeff  p_tire=250e3 Pa  alpha=-0.003  beta=0.97  coeff_a=84e-4  coeff_b=6.2e-4 s/m  coeff_c=1.6e-4 s^2/m^2  p_tire0=240e3 Pa  fz0_resistance=4000 N  vH0=16 m/s  q_Sy=[.0082, 0, .0014, .001, 0, 0, 1.08, -.5]  v_thr=0.001 m/s  enable_scaling_coefficients=false  lfzO=1  lcx=1  lmux=1  lex=1  lkx=1  lhx=1  lvx=1  lmy=1  model_compliance=sdl.enum.compliance.off  stiffness=1e6 N/m  damping=1000 N*s/m  model_inertia=sdl.enum.model_inertia.on  inertia=1 kg*m^2  initial_velocity=0 rad/s  vxlow=0.1*(0.1) m/s  v_tr_thr=0.1*(0.1*(0.1)) m/s  kpumin=-1e5  kpumax=1e5
  Simulink-PS Converter3 : nesl_utility/Simulink-PS Converter  PhysicalDomain=network_engine_domain  SubClassName=ps_input  LeftPortType=input  RightPortType=output  PseudoPeriodic=off  Frequencies=[]  NoiseDistribution=none  NoiseParameters=[]  Unit=Pa  AffineConversion=off  FilteringAndDerivatives=zero  SimscapeFilterOrder=1  InputFilterTimeConstant=0.001  UdotUserProvided=1
  N_FL : PMIOPort  Side=Left
  H_FL : PMIOPort  Port=2  Side=Right
  T_FL : PMIOPort  Port=3  Side=Left
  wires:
  [Brake] -> Simulink-PS Converter3/1
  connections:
  Disc Brake1/LConn2 -- FL Tire/LConn2 -- T_FL/RConn1
  FL Tire/LConn1 -- N_FL/RConn1
  Simulink-PS Converter3/RConn1 -- Disc Brake1/LConn1
  FL Tire/RConn2 -- H_FL/RConn1

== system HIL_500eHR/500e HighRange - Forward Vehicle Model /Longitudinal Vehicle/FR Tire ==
  Disc Brake1 : sdl_lib/Brakes & Detents/Rotational/Disc Brake  r_mean=150 mm  bore=10 mm  n_pads=2  thermal_port=simscape.enum.thermaleffects.omit  mu_static=0.9  mu_coulomb=0.7  temperature_TLU=[280, 300, 320] K  mu_static_TLU=[.9, .8, .7]  mu_coulomb_TLU=[.8, .7, .6]  brkwy_vel=0.1 rad/s  visc_coef=.001 N*m/(rad/s)  enable_faults=simscape.enum.onoff.off  faulted_pressure=0 bar  external_fault=simscape.enum.onoff.off  temporal_fault=simscape.enum.onoff.off  fault_time=5 s  report_fault=simscape.enum.assert.action.none  thermal_mass=50 kJ/K  temperature_specify=off  temperature_priority=High  temperature=300 K  temperature_nominal_specify=off  temperature_nominal_unit=K  temperature_nominal_value=1
  FR Tire : sdl_lib/Tires & Vehicles/Tire (Magic Formula)  parameterization=sdl.enum.magic_tire_model.peak  F_z1=vehicle.mass*9.81/4 N  F_x1=3500 N  kappa1=10  B_m=14.2649  C_m=2.9817  D_m=0.7035  E_m=1.5923  fz0=4000 N  p_Cx=1.685  p_Dx=[1.21, -.037]  p_Ex=[.344, .095, -.02, 0]  p_Kx=[21.51, -.163, .245]  p_Hx=[-.002, .002]  p_Vx=[0, 0]  rolling_radius_model=sdl.enum.RollingRadiusParameterization.Constant  r_e=vehicle.tireRollingRadius m  r_0=0.3 m  breff=8.39  dreff=0.26  freff=0.074  q_re0=0.99  q_v1=0.008  longvl=17 m/s  cz=5e5 N/m  model_resistance=simscape.enum.onoff.on  resistance_model=sdl.enum.rollingResistanceParameterization.constant  coeff=vehicle.tireRRcoeff  p_tire=250e3 Pa  alpha=-0.003  beta=0.97  coeff_a=84e-4  coeff_b=6.2e-4 s/m  coeff_c=1.6e-4 s^2/m^2  p_tire0=240e3 Pa  fz0_resistance=4000 N  vH0=16 m/s  q_Sy=[.0082, 0, .0014, .001, 0, 0, 1.08, -.5]  v_thr=0.001 m/s  enable_scaling_coefficients=false  lfzO=1  lcx=1  lmux=1  lex=1  lkx=1  lhx=1  lvx=1  lmy=1  model_compliance=sdl.enum.compliance.off  stiffness=1e6 N/m  damping=1000 N*s/m  model_inertia=sdl.enum.model_inertia.on  inertia=1 kg*m^2  initial_velocity=0 rad/s  vxlow=0.1*(0.1) m/s  v_tr_thr=0.1*(0.1*(0.1)) m/s  kpumin=-1e5  kpumax=1e5
  Simulink-PS Converter1 : nesl_utility/Simulink-PS Converter  PhysicalDomain=network_engine_domain  SubClassName=ps_input  LeftPortType=input  RightPortType=output  PseudoPeriodic=off  Frequencies=[]  NoiseDistribution=none  NoiseParameters=[]  Unit=Pa  AffineConversion=off  FilteringAndDerivatives=zero  SimscapeFilterOrder=1  InputFilterTimeConstant=0.001  UdotUserProvided=1
  H_RR : PMIOPort  Side=Right
  T_RR : PMIOPort  Port=2  Side=Left
  N_RR : PMIOPort  Port=3  Side=Left
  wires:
  [Brake] -> Simulink-PS Converter1/1
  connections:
  FR Tire/LConn1 -- N_RR/RConn1
  T_RR/RConn1 -- Disc Brake1/LConn2 -- FR Tire/LConn2
  Simulink-PS Converter1/RConn1 -- Disc Brake1/LConn1
  FR Tire/RConn2 -- H_RR/RConn1

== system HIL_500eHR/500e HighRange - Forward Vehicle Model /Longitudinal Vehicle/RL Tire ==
  Disc Brake : sdl_lib/Brakes & Detents/Rotational/Disc Brake  r_mean=150 mm  bore=10 mm  n_pads=2  thermal_port=simscape.enum.thermaleffects.omit  mu_static=0.9  mu_coulomb=0.7  temperature_TLU=[280, 300, 320] K  mu_static_TLU=[.9, .8, .7]  mu_coulomb_TLU=[.8, .7, .6]  brkwy_vel=0.1 rad/s  visc_coef=.001 N*m/(rad/s)  enable_faults=simscape.enum.onoff.off  faulted_pressure=0 bar  external_fault=simscape.enum.onoff.off  temporal_fault=simscape.enum.onoff.off  fault_time=5 s  report_fault=simscape.enum.assert.action.none  thermal_mass=50 kJ/K  temperature_specify=off  temperature_priority=High  temperature=300 K  temperature_nominal_specify=off  temperature_nominal_unit=K  temperature_nominal_value=1
  RL Tire : sdl_lib/Tires & Vehicles/Tire (Magic Formula)  parameterization=sdl.enum.magic_tire_model.peak  F_z1=vehicle.mass*9.81/4 N  F_x1=3500 N  kappa1=10  B_m=14.2649  C_m=2.9817  D_m=0.7035  E_m=1.5923  fz0=4000 N  p_Cx=1.685  p_Dx=[1.21, -.037]  p_Ex=[.344, .095, -.02, 0]  p_Kx=[21.51, -.163, .245]  p_Hx=[-.002, .002]  p_Vx=[0, 0]  rolling_radius_model=sdl.enum.RollingRadiusParameterization.Constant  r_e=vehicle.tireRollingRadius m  r_0=0.3 m  breff=8.39  dreff=0.26  freff=0.074  q_re0=0.99  q_v1=0.008  longvl=17 m/s  cz=5e5 N/m  model_resistance=simscape.enum.onoff.on  resistance_model=sdl.enum.rollingResistanceParameterization.constant  coeff=vehicle.tireRRcoeff  p_tire=250e3 Pa  alpha=-0.003  beta=0.97  coeff_a=84e-4  coeff_b=6.2e-4 s/m  coeff_c=1.6e-4 s^2/m^2  p_tire0=240e3 Pa  fz0_resistance=4000 N  vH0=16 m/s  q_Sy=[.0082, 0, .0014, .001, 0, 0, 1.08, -.5]  v_thr=0.001 m/s  enable_scaling_coefficients=false  lfzO=1  lcx=1  lmux=1  lex=1  lkx=1  lhx=1  lvx=1  lmy=1  model_compliance=sdl.enum.compliance.off  stiffness=1e6 N/m  damping=1000 N*s/m  model_inertia=sdl.enum.model_inertia.on  inertia=1 kg*m^2  initial_velocity=0 rad/s  vxlow=0.1*(0.1) m/s  v_tr_thr=0.1*(0.1*(0.1)) m/s  kpumin=-1e5  kpumax=1e5
  Simulink-PS Converter : nesl_utility/Simulink-PS Converter  PhysicalDomain=network_engine_domain  SubClassName=ps_input  LeftPortType=input  RightPortType=output  PseudoPeriodic=off  Frequencies=[]  NoiseDistribution=none  NoiseParameters=[]  Unit=Pa  AffineConversion=off  FilteringAndDerivatives=zero  SimscapeFilterOrder=1  InputFilterTimeConstant=0.001  UdotUserProvided=1
  N_RL : PMIOPort  Side=Left
  H_RL : PMIOPort  Port=2  Side=Right
  T_RL : PMIOPort  Port=3  Side=Left
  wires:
  [Brake] -> Simulink-PS Converter/1
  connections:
  RL Tire/RConn2 -- H_RL/RConn1
  RL Tire/LConn1 -- N_RL/RConn1
  T_RL/RConn1 -- RL Tire/LConn2 -- Disc Brake/LConn2
  Simulink-PS Converter/RConn1 -- Disc Brake/LConn1

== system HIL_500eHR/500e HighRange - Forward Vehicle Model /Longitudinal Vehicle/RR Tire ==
  Disc Brake : sdl_lib/Brakes & Detents/Rotational/Disc Brake  r_mean=150 mm  bore=10 mm  n_pads=2  thermal_port=simscape.enum.thermaleffects.omit  mu_static=0.9  mu_coulomb=0.7  temperature_TLU=[280, 300, 320] K  mu_static_TLU=[.9, .8, .7]  mu_coulomb_TLU=[.8, .7, .6]  brkwy_vel=0.1 rad/s  visc_coef=.001 N*m/(rad/s)  enable_faults=simscape.enum.onoff.off  faulted_pressure=0 bar  external_fault=simscape.enum.onoff.off  temporal_fault=simscape.enum.onoff.off  fault_time=5 s  report_fault=simscape.enum.assert.action.none  thermal_mass=50 kJ/K  temperature_specify=off  temperature_priority=High  temperature=300 K  temperature_nominal_specify=off  temperature_nominal_unit=K  temperature_nominal_value=1
  RR Tire : sdl_lib/Tires & Vehicles/Tire (Magic Formula)  parameterization=sdl.enum.magic_tire_model.peak  F_z1=vehicle.mass*9.81/4 N  F_x1=3500 N  kappa1=10  B_m=14.2649  C_m=2.9817  D_m=0.7035  E_m=1.5923  fz0=4000 N  p_Cx=1.685  p_Dx=[1.21, -.037]  p_Ex=[.344, .095, -.02, 0]  p_Kx=[21.51, -.163, .245]  p_Hx=[-.002, .002]  p_Vx=[0, 0]  rolling_radius_model=sdl.enum.RollingRadiusParameterization.Constant  r_e=vehicle.tireRollingRadius m  r_0=0.3 m  breff=8.39  dreff=0.26  freff=0.074  q_re0=0.99  q_v1=0.008  longvl=17 m/s  cz=5e5 N/m  model_resistance=simscape.enum.onoff.on  resistance_model=sdl.enum.rollingResistanceParameterization.constant  coeff=vehicle.tireRRcoeff  p_tire=250e3 Pa  alpha=-0.003  beta=0.97  coeff_a=84e-4  coeff_b=6.2e-4 s/m  coeff_c=1.6e-4 s^2/m^2  p_tire0=240e3 Pa  fz0_resistance=4000 N  vH0=16 m/s  q_Sy=[.0082, 0, .0014, .001, 0, 0, 1.08, -.5]  v_thr=0.001 m/s  enable_scaling_coefficients=false  lfzO=1  lcx=1  lmux=1  lex=1  lkx=1  lhx=1  lvx=1  lmy=1  model_compliance=sdl.enum.compliance.off  stiffness=1e6 N/m  damping=1000 N*s/m  model_inertia=sdl.enum.model_inertia.on  inertia=1 kg*m^2  initial_velocity=0 rad/s  vxlow=0.1*(0.1) m/s  v_tr_thr=0.1*(0.1*(0.1)) m/s  kpumin=-1e5  kpumax=1e5
  Simulink-PS Converter : nesl_utility/Simulink-PS Converter  PhysicalDomain=network_engine_domain  SubClassName=ps_input  LeftPortType=input  RightPortType=output  PseudoPeriodic=off  Frequencies=[]  NoiseDistribution=none  NoiseParameters=[]  Unit=Pa  AffineConversion=off  FilteringAndDerivatives=zero  SimscapeFilterOrder=1  InputFilterTimeConstant=0.001  UdotUserProvided=1
  H_RR : PMIOPort  Side=Right
  T_RR : PMIOPort  Port=2  Side=Left
  N_RR : PMIOPort  Port=3  Side=Left
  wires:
  [Brake] -> Simulink-PS Converter/1
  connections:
  RR Tire/LConn1 -- N_RR/RConn1
  T_RR/RConn1 -- RR Tire/LConn2 -- Disc Brake/LConn2
  Simulink-PS Converter/RConn1 -- Disc Brake/LConn1
  RR Tire/RConn2 -- H_RR/RConn1
